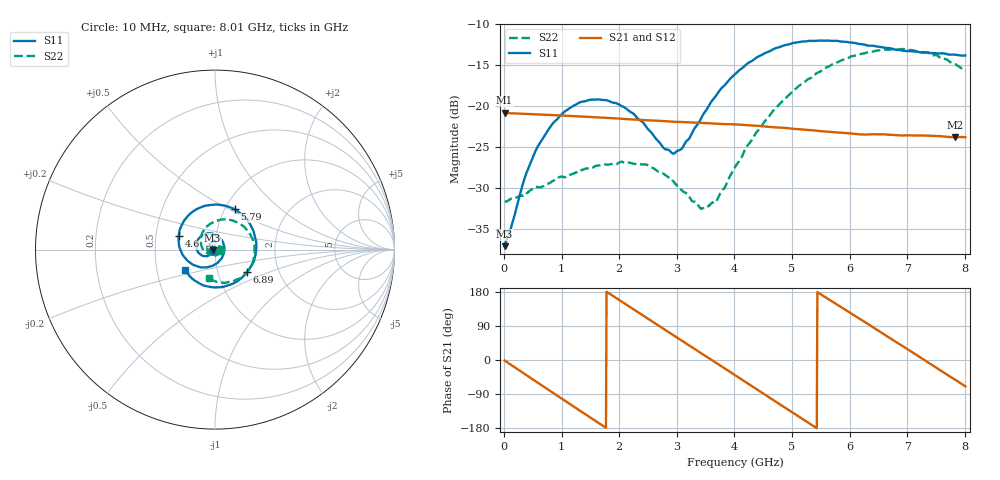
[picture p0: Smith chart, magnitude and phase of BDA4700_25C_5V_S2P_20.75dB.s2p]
!Agilent Technologies,E5071B,MY42404982,A.09.10
!Date: Mon Oct 20 13:36:47 2025
!Data & Calibration Information:
!Freq	S11:SOLT2(ON)	S21:SOLT2(ON)	S12:SOLT2(ON)	S22:SOLT2(ON)
# Hz S RI R 50
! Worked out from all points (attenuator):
!   801 points, 10 MHz to 8.01 GHz, reference 50 ohm
!   highest |S21| = -20.83 dB at 10 MHz (marker M1); lowest = -23.8 dB at 7.83 GHz (marker M2)
!   lowest |S11| = -37.1 dB at 10 MHz (marker M3), VSWR 1.03, Z = 48.6 - j0.139 ohm
!   |S11| at or under -10 dB: start of sweep to end of sweep
!   |S22| runs from -32.6 to -13.0 dB; largest |S21 - S12| = 0.00074
!   S11 on the Smith chart (normalised r, x): 10 MHz: 0.97, -0.00; 4.6 GHz: 0.66, +0.10; 5.79 GHz: 1.11, +0.53; 6.89 GHz: 1.38, -0.36; 8.01 GHz: 0.70, -0.17
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1e7  -0.0138 -0.00143  0.0908 -0.00193  0.0908 -0.00203  0.0261 -0.000822
3.7e8  -0.0255 -0.027  0.0704 -0.0552  0.0704 -0.0552  0.0216 -0.0189
5.8e8  -0.0426 -0.0363  0.0452 -0.0764  0.0452 -0.0764  0.014 -0.0287
9.9e8  -0.0846 -0.0246  -0.0164 -0.0859  -0.0164 -0.0859  -0.0142 -0.034
1.35e9  -0.105 0.0156  -0.063 -0.0588  -0.063 -0.0588  -0.0364 -0.0177
1.76e9  -0.0829 0.07  -0.0846 -0.0029  -0.0847 -0.00291  -0.0421 0.0126
2.07e9  -0.0397 0.0905  -0.073 0.0403  -0.0731 0.0403  -0.03 0.0339
2.68e9  0.0442 0.0417  -0.00119 0.0811  -0.00118 0.0811  0.0138 0.0371
2.98e9  0.0504 -0.0139  0.0382 0.0702  0.0383 0.0702  0.0266 0.0201
3.44e9  -0.00629 -0.0864  0.0757 0.0219  0.0757 0.0219  0.0182 -0.0149
3.69e9  -0.0618 -0.0992  0.0771 -0.0113  0.0771 -0.0116  -0.00019 -0.0262
4.01e9  -0.1375 -0.0741  0.0591 -0.0495  0.0591 -0.0495  -0.0331 -0.0259
4.6e9  -0.2017 0.075  -0.011 -0.0737  -0.0109 -0.0738  -0.0786 0.0356
4.93e9  -0.1638 0.1721  -0.0478 -0.0552  -0.0478 -0.0555  -0.0716 0.0904
5.35e9  -0.0447 0.246  -0.0703 -0.00979  -0.0704 -0.01  -0.0151 0.1494
5.79e9  0.109 0.225  -0.0566 0.0393  -0.0565 0.0394  0.0828 0.1653
6.23e9  0.2132 0.1055  -0.0154 0.0651  -0.0148 0.0653  0.178 0.1093
6.68e9  0.218 -0.0583  0.0336 0.0576  0.0338 0.0576  0.2203 -0.00267
6.89e9  0.1795 -0.1255  0.0509 0.042  0.0511 0.0418  0.2135 -0.0615
7.35e9  0.0357 -0.2094  0.0655 -0.00581  0.0656 -0.00594  0.1383 -0.1607
7.83e9  -0.1263 -0.1627  0.0398 -0.0505  0.0398 -0.0506  0.0107 -0.1803
8.01e9  -0.1674 -0.1158  0.0225 -0.0603  0.0226 -0.0604  -0.0323 -0.1601
